(* Logix 5000 Program export Yaskawa_Ladder; software revision 17.00 *)

TYPE YaskawaParameters :   // DRIVE CONFIGURATION
STRUCT
   Parameters : DINT[43];   // DRIVE PARAMETERS
   Monitor : INT[43];   // DRIVE MONITOR VALUES
   CommsPath : STRING;   // COMMUNICATION PATH
   Slot : DINT;   // Slot # entered by HMI
   GetValues : BOOL;   // GET PARAMETER VALUES
   SetValues : BOOL;   // SET PARAMETER VALUES
   SetPath : BOOL;   // SET COMMUNICATIONS PATH
   MSG_Value : INT;   // INDIVIDUAL PARAMETER VALUE
   FinalFIFO_Pos : INT;   // FIFO LENGTH
   MSG_Attribute : INT;   // MESSAGE ATTRIBUTE CONFIGURATION
   MSG_Class : INT;   // MESSAGE CLASS CONFIGURATION
   MSG_Instance : INT;   // MESSAGE INSTANCE CONFIGURATION
   ONS : INT;   // ONE-SHOTS
   AttributeArray : INT[43];   // ATTRIBUTE ARRAY
   ClassArray : INT[43];   // CLASS ARRAY
   InstanceArray : INT[43];   // INSTANCE ARRAY
   CycleTimer : TIMER[7];   // MESSAGE TIMERS
   FIFO : CONTROL;   // PARAMETER FIFO
   Update : BOOL;   // GET MONITOR VALUES
   FIFO_Monitor : CONTROL;   // MONITOR FIFO
   MonitorMSG_Value : INT;   // INDIVIDUAL MONITOR VALUE
   Monitor_ClassArray : INT[43];   // MONITOR CLASS ARRAY
   Monitor_AttributeArray : INT[43];   // MONITOR ATTRIBUTE ARRAY
   Monitor_InstanceArray : INT[43];   // MONITOR INSTANCE ARRAY
   Monitor_MSG_Attribute : INT;   // MONITOR MESSAGE ATTRIBUTE CONFIGURATION
   Monitor_MSG_Class : INT;   // MONITOR MESSAGE CLASS CONFIGURATION
   Monitor_MSG_Instance : INT;   // MONITOR MESSAGE INSTANCE CONFIGURATION
   AB_CommsPath : STRING[17];   // AB SLOT CONFIG
   IP_StringCount : STRING[16];   // Indicates variable to use in path for given IP string character count
   MSG_CommsPath : STRING;   // TOTAL COMM PATH FOR MESSAGE INST
   counter : COUNTER[4];
   A : STRING;   // Constant string value A
   ASCII_Extract : DINT;
   B : STRING;   // Constant string value B
   C : STRING;   // Constant string value C
   Convert_Start : BOOL;   // Used to begin the convert of hex string to decimal value
   Current_Index : DINT;
   D : STRING;   // Constant string value D
   DINT : DINT;   // Holds value passed as input parameter from main routine
   E : STRING;   // Constant string value E
   EMPTY : STRING;   // Empty string used to reset the final string value before concatenation
   F : STRING;   // Constant string value F
   Hex_Entry_Flag : BOOL[32];   // Bit for HMI entry to trigger conversion of hex string to decimal
   Hex_OpEntry_Read : STRING[37];   // Array to hold hex string values for display on HMI
   Hex_OpEntry_Write : STRING[14];   // Array to hold hex string values entered by HMI to be converted
   Hex_Read_Placeholder : DINT;   // Placeholder to retrieve hex string for HMI display
   HTD_Number : DINT;
   HTD_String : STRING;
   J : DINT;   // Used to make a FOR/NEXT loop
   NUMBER : DINT;
   Partial_DINT : DINT[8];   // Holds individual parts from the original DINT values
   Partial_STRING : STRING[8];   // Holds individual from the original DINT in string format
   STRING : STRING;   // Contains the final value
   tempstring : STRING[4];   // Temporary string to concatinate communication path to message instructions
   Current_Fault : STRING;
   Last_Fault : STRING;
   Fault_Codes : STRING[775];
   K : DINT;
   Auto_Update : BOOL;   // Bit to turn on or off auto update of Monitor parameters
   MSGPath_Ending : STRING;   // Always $00
END_STRUCT
END_TYPE

VAR_GLOBAL   (* controller tags *)
   YaskawaMSG_Write : MESSAGE;   // YASKAWA DRIVE PARAMTER WRITE
        MessageParameters(MessageType := CIP Generic, RequestedLength := 2, ConnectedFlag := 2, ConnectionPath := test, 2, 192.165.1.165, ServiceCode := 16#0010, LocalElement := Yaskawa.MSG_Value)
   Yaskawa : YaskawaParameters;
        .PARAMETERS[1]   // DRIVE ENTRY PARAMETER
        .PARAMETERS[2]   // B1-01 - FREQUENCY REFERENCE SELECTION 1
        .PARAMETERS[3]   // B1-02 - RUN COMMAND SELECTION 1
        .PARAMETERS[4]   // C1-01 - ACCELERATION TIME
        .PARAMETERS[5]   // C1-02 - DECELERATION TIME
        .PARAMETERS[6]   // D1-01 - FREQUENCY REFERENCE 1
        .PARAMETERS[7]   // D1-02 - FREQUENCY REFERENCE 2
        .PARAMETERS[8]   // D1-03 - FREQUENCY REFERENCE 3
        .PARAMETERS[9]   // D1-04 - FREQUENCY REFERENCE 4
        .PARAMETERS[10]   // D1-17 - JOG REFERENCE
        .PARAMETERS[11]   // E1-01 - INPUT VOLTAGE
        .PARAMETERS[12]   // E1-04 - MAXIMUM OUTPUT FREQUENCY
        .PARAMETERS[13]   // E1-05 - MAXIMUM OUTPUT VOLTAGE
        .PARAMETERS[14]   // E1-06 - BASE FREQUENCY
        .PARAMETERS[15]   // E1-13 - BASE VOLTAGE
        .PARAMETERS[16]   // E2-01 - MOTOR RATED CURRENT
        .PARAMETERS[17]   // E2-02 - MOTOR RATED SLIP
        .PARAMETERS[18]   // E2-03 - MOTOR NO-LOAD CURRENT
        .PARAMETERS[19]   // E2-04 - NUMBER OF MOTOR POLES
        .PARAMETERS[20]   // E2-05 - MOTOR LINE TO LINE RESISTANCE
        .PARAMETERS[21]   // E2-11 - MOTOR RATED POWER
        .PARAMETERS[22]   // H1-01 - MULTI-FUNCTION INPUT S1
        .PARAMETERS[23]   // H1-02 - MULTI-FUNCTION INPUT S2
        .PARAMETERS[24]   // H1-03 - MULTI-FUNCTION INPUT S3
        .PARAMETERS[25]   // H1-04 - MULTI-FUNCTION INPUT S4
        .PARAMETERS[26]   // H1-05 - MULTI-FUNCTION INPUT S5
        .PARAMETERS[27]   // H1-06 - MULTI-FUNCTION INPUT S6
        .PARAMETERS[28]   // H1-07 - MULTI-FUNCTION INPUT S7
        .PARAMETERS[29]   // H1-08 - MULTI-FUNCTION INPUT S8
        .PARAMETERS[30]   // H2-01 - MULTI FUNCTION OUTPUT M1-M2
        .PARAMETERS[31]   // H2-02 - MULTI-FUNCTION OUTPUT M3-M4
        .PARAMETERS[32]   // H2-03 - MULTI FUNCTION OUTPUT M5-M6
        .PARAMETERS[33]   // H3-02 - TERMINAL A1 FUNCTION SELECTION
        .PARAMETERS[34]   // H3-06 - TERMINAL A3 FUNCTION SELECTION
        .PARAMETERS[35]   // H3-10 - TERMINAL A2 FUNCTION SELECTION
        .PARAMETERS[36]   // H4-01 - MULTI-FUNCTION ANALOG OUTPUT SELECTION (FM)
        .PARAMETERS[37]   // H4-04 - MULTI-FUNCTION ANALOG OUTPUT (AM)
        .PARAMETERS[38]   // L1-01 - MOTOR OVERLOAD PROTECTION SELECTION
        .PARAMETERS[39]   // L5-01 - NUMBER OF AUTO-RESTART ATTEMPTS
        .PARAMETERS[40]   // A1-02 - CONTROL METHOD
        .PARAMETERS[41]   // A1-06 - APPLICATION PRESETS
        .MONITOR[1]   // U1-02 - FREQUENCY OUTPUT
        .MONITOR[2]   // U1-03 - OUTPUT CURRENT
        .MONITOR[3]   // U1-05 - MOTOR SPEED
        .MONITOR[4]   // U1-06 - OUTPUT VOLTAGE
        .MONITOR[5]   // U1-07 - DC BUS VOLTAGE
        .MONITOR[6]   // U1-08 - OUTPUT POWER
        .MONITOR[7]   // U1-09 - TORQUE REFERENCE
        .MONITOR[8]   // U1-10 - INPUT TERMINAL STATUS
        .MONITOR[9]   // U1-11 - OUTPUT TERMINAL STATUS
        .MONITOR[10]   // U1-12 - DRIVE STATUS
        .MONITOR[11]   // U1-13 - TERMINAL A1 INPUT LEVEL
        .MONITOR[12]   // U1-14 - TERMINAL A2 INPUT LEVEL
        .MONITOR[13]   // U1-15 - TERMINAL A3 INPUT LEVEL
        .MONITOR[14]   // U2-01 - CURRENT FAULT
        .MONITOR[15]   // U2-02 - LAST FAULT
        .MONITOR[16]   // U2-03 - FREQUENCY REFERENCE AT PREVIOUS FAULT
        .MONITOR[17]   // U2-04 - OUTPUT FREQUENCY AT PREVIOUS FAULT
        .MONITOR[18]   // U2-05 - OUTPUT AT PREVIOUS FAULT
        .MONITOR[19]   // U2-06 - MOTOR SPEED AT PREVIOUS FAULT
        .MONITOR[20]   // U2-07 - OUTPUT VOLTAGE AT PREVIOUS FAULT
        .MONITOR[21]   // U2-08 - DC BUS VOLTAGE AT PREVIOUS FAULT
        .MONITOR[22]   // U2-09 - OUTPUT POWER AT PREVIOUS FAULT
        .MONITOR[23]   // U2-10 - TORQUE REFERENCE AT PREVIOUS FAULT
        .MONITOR[24]   // U2-11 - INPUT TERMINAL STATUS AT PREVIOUS FAULT
        .MONITOR[25]   // U2-12 - OUTPUT TERMINAL STATUS AT PREVIOUS FAULT
        .MONITOR[26]   // U2-13 - DRIVE OPERATION STATUS AT PREVIOUS FAULT
        .MONITOR[27]   // U2-14 - CUMULATIVE OPERATION TIME AT PREVIOUS FAULT
        .MONITOR[28]   // U1-01 - FREQUENCY REFERENCE
   YaskawaMSG_Monitor : MESSAGE;   // YASKAWA DRIVE MONITOR READ
        MessageParameters(MessageType := CIP Generic, ConnectedFlag := 2, ConnectionPath := test, 2, 192.165.1.165, ServiceCode := 16#000e, DestinationTag := Yaskawa.MonitorMSG_Value)
   YaskawaMSG_Read : MESSAGE;   // YASKAWA DRIVE PARAMETER READ
        MessageParameters(MessageType := CIP Generic, ConnectedFlag := 2, ConnectionPath := test, 2, 192.165.1.165, ServiceCode := 16#000e, DestinationTag := Yaskawa.MSG_Value)
END_VAR

PROGRAM Yaskawa_Ladder   (* main routine Yaskawa_Parameters *)

ROUTINE Yaskawa_Monitor   (* ladder *)
// Controls collecting U parameters for monitoring.
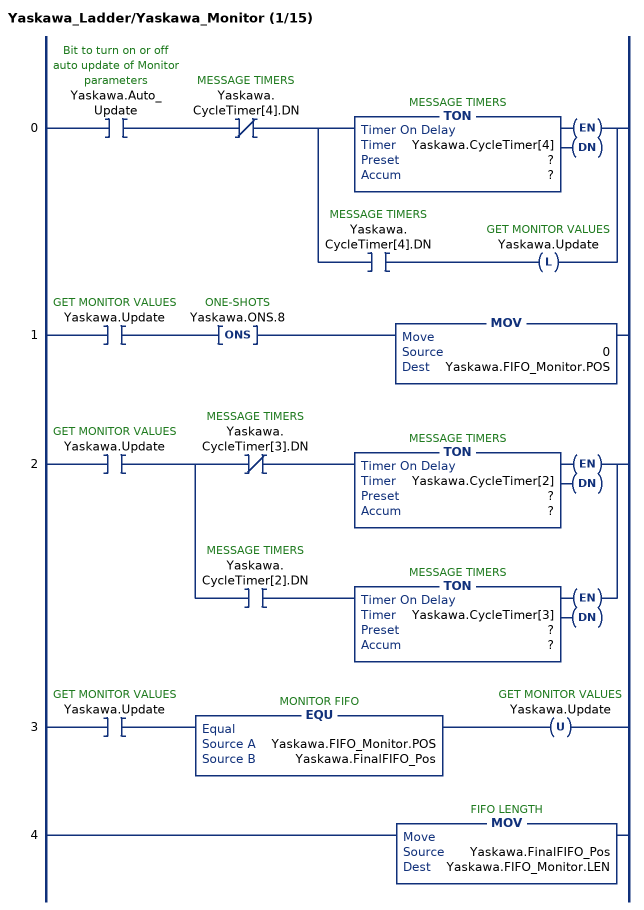
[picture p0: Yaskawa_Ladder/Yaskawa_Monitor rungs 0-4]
   0: XIC(Yaskawa.Auto_Update)XIO(Yaskawa.CycleTimer[4].DN)[TON(Yaskawa.CycleTimer[4],?,?) ,XIC(Yaskawa.CycleTimer[4].DN) OTL(Yaskawa.Update) ];
   1: XIC(Yaskawa.Update)ONS(Yaskawa.ONS.8)MOV(0,Yaskawa.FIFO_Monitor.POS);
   2: XIC(Yaskawa.Update)[XIO(Yaskawa.CycleTimer[3].DN) TON(Yaskawa.CycleTimer[2],?,?) ,XIC(Yaskawa.CycleTimer[2].DN) TON(Yaskawa.CycleTimer[3],?,?) ];
   3: XIC(Yaskawa.Update)EQU(Yaskawa.FIFO_Monitor.POS,Yaskawa.FinalFIFO_Pos)OTU(Yaskawa.Update);
   4: MOV(Yaskawa.FinalFIFO_Pos,Yaskawa.FIFO_Monitor.LEN);
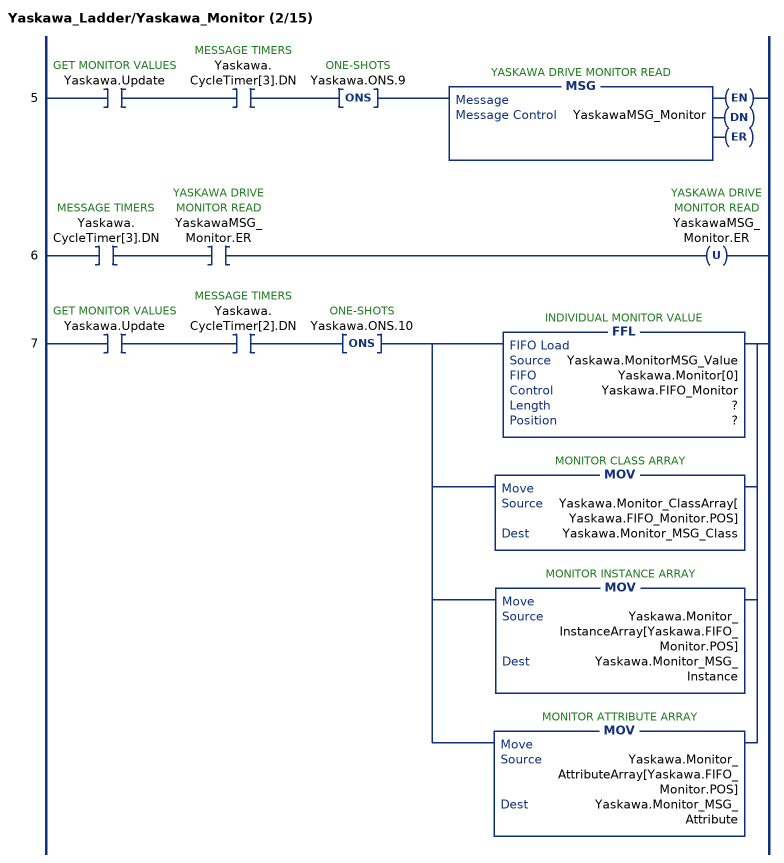
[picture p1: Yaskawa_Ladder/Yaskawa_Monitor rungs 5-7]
   5: XIC(Yaskawa.Update)XIC(Yaskawa.CycleTimer[3].DN)ONS(Yaskawa.ONS.9)MSG(YaskawaMSG_Monitor);
   6: XIC(Yaskawa.CycleTimer[3].DN)XIC(YaskawaMSG_Monitor.ER)OTU(YaskawaMSG_Monitor.ER);
   7: XIC(Yaskawa.Update)XIC(Yaskawa.CycleTimer[2].DN)ONS(Yaskawa.ONS.10)[FFL(Yaskawa.MonitorMSG_Value,Yaskawa.Monitor[0],Yaskawa.FIFO_Monitor,?,?) ,MOV(Yaskawa.Monitor_ClassArray[Yaskawa.FIFO_Monitor.POS],Yaskawa.Monitor_MSG_Class) ,MOV(Yaskawa.Monitor_InstanceArray[Yaskawa.FIFO_Monitor.POS],Yaskawa.Monitor_MSG_Instance) ,MOV(Yaskawa.Monitor_AttributeArray[Yaskawa.FIFO_Monitor.POS],Yaskawa.Monitor_MSG_Attribute) ];
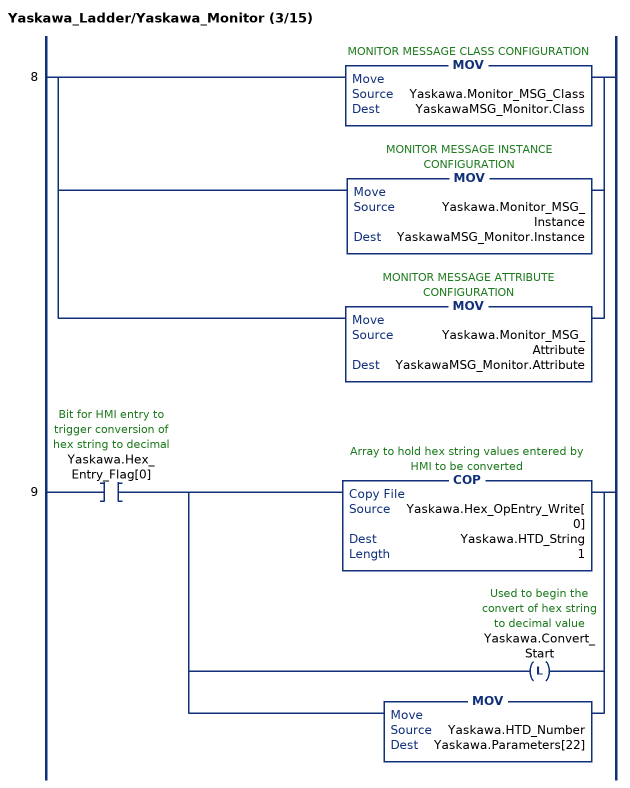
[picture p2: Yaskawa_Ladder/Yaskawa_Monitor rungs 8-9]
   8: [MOV(Yaskawa.Monitor_MSG_Class,YaskawaMSG_Monitor.Class) ,MOV(Yaskawa.Monitor_MSG_Instance,YaskawaMSG_Monitor.Instance) ,MOV(Yaskawa.Monitor_MSG_Attribute,YaskawaMSG_Monitor.Attribute) ];
   9: XIC(Yaskawa.Hex_Entry_Flag[0])[COP(Yaskawa.Hex_OpEntry_Write[0],Yaskawa.HTD_String,1) ,OTL(Yaskawa.Convert_Start) ,MOV(Yaskawa.HTD_Number,Yaskawa.Parameters[22]) ];
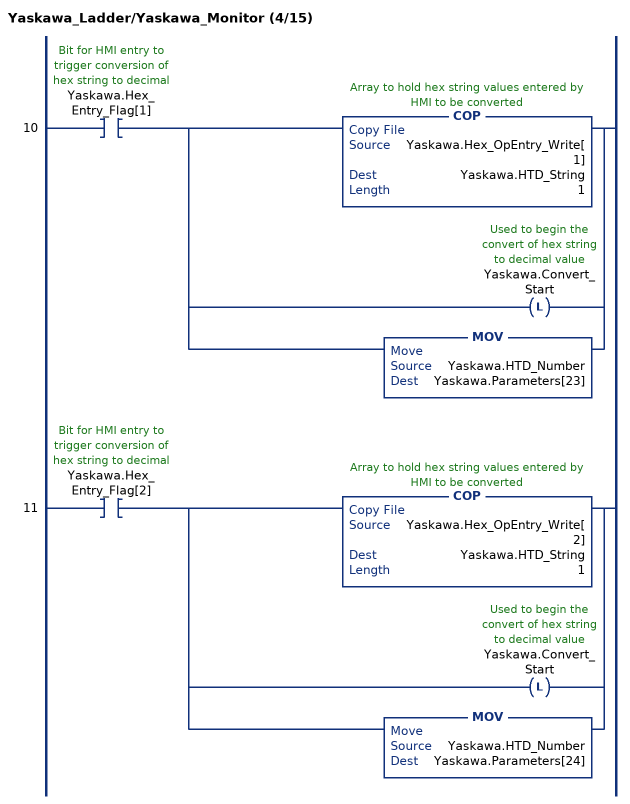
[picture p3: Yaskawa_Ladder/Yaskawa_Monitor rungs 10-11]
   10: XIC(Yaskawa.Hex_Entry_Flag[1])[COP(Yaskawa.Hex_OpEntry_Write[1],Yaskawa.HTD_String,1) ,OTL(Yaskawa.Convert_Start) ,MOV(Yaskawa.HTD_Number,Yaskawa.Parameters[23]) ];
   11: XIC(Yaskawa.Hex_Entry_Flag[2])[COP(Yaskawa.Hex_OpEntry_Write[2],Yaskawa.HTD_String,1) ,OTL(Yaskawa.Convert_Start) ,MOV(Yaskawa.HTD_Number,Yaskawa.Parameters[24]) ];
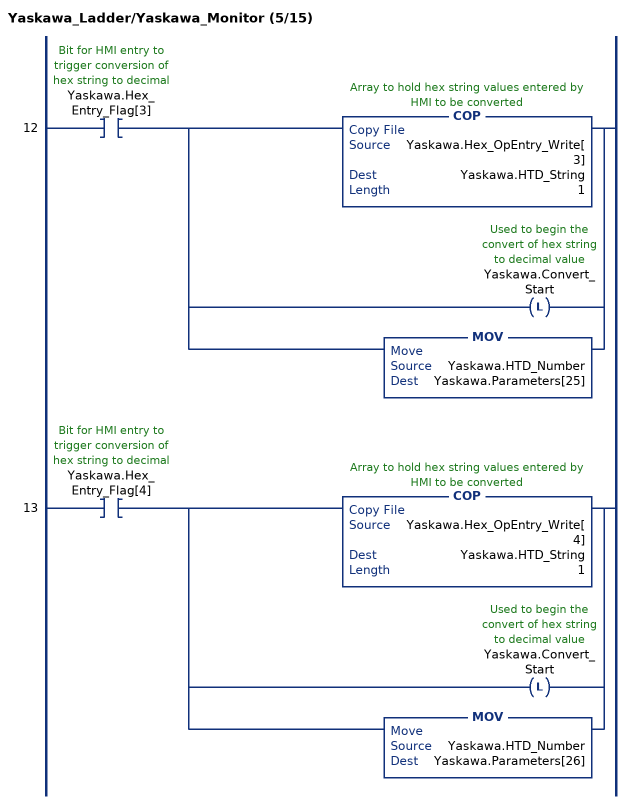
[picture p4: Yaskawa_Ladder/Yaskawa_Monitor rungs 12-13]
   12: XIC(Yaskawa.Hex_Entry_Flag[3])[COP(Yaskawa.Hex_OpEntry_Write[3],Yaskawa.HTD_String,1) ,OTL(Yaskawa.Convert_Start) ,MOV(Yaskawa.HTD_Number,Yaskawa.Parameters[25]) ];
   13: XIC(Yaskawa.Hex_Entry_Flag[4])[COP(Yaskawa.Hex_OpEntry_Write[4],Yaskawa.HTD_String,1) ,OTL(Yaskawa.Convert_Start) ,MOV(Yaskawa.HTD_Number,Yaskawa.Parameters[26]) ];
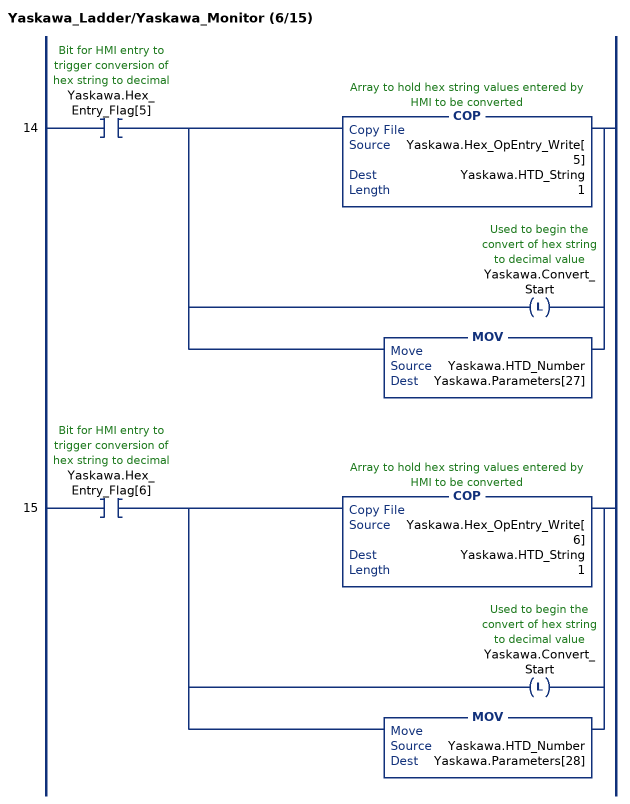
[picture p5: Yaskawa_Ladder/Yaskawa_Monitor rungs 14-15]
   14: XIC(Yaskawa.Hex_Entry_Flag[5])[COP(Yaskawa.Hex_OpEntry_Write[5],Yaskawa.HTD_String,1) ,OTL(Yaskawa.Convert_Start) ,MOV(Yaskawa.HTD_Number,Yaskawa.Parameters[27]) ];
   15: XIC(Yaskawa.Hex_Entry_Flag[6])[COP(Yaskawa.Hex_OpEntry_Write[6],Yaskawa.HTD_String,1) ,OTL(Yaskawa.Convert_Start) ,MOV(Yaskawa.HTD_Number,Yaskawa.Parameters[28]) ];
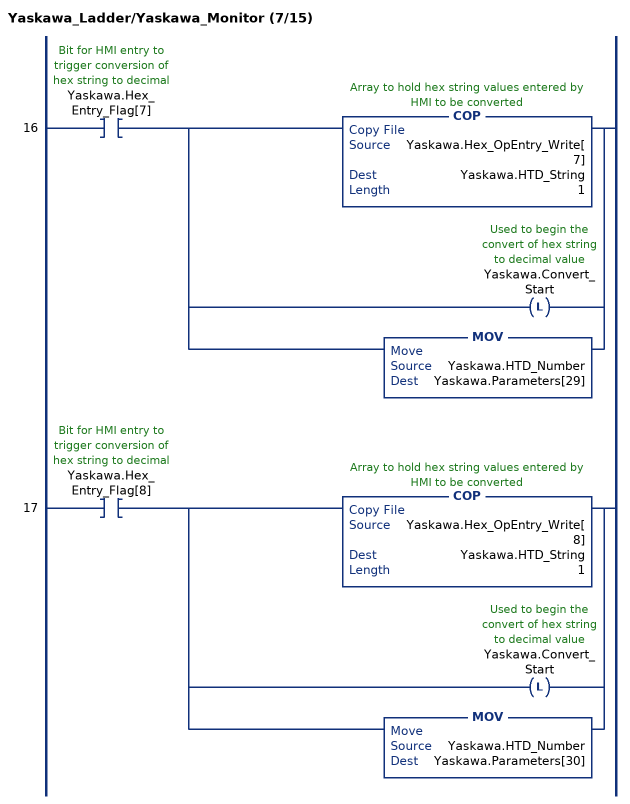
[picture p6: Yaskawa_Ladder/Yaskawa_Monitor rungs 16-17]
   16: XIC(Yaskawa.Hex_Entry_Flag[7])[COP(Yaskawa.Hex_OpEntry_Write[7],Yaskawa.HTD_String,1) ,OTL(Yaskawa.Convert_Start) ,MOV(Yaskawa.HTD_Number,Yaskawa.Parameters[29]) ];
   17: XIC(Yaskawa.Hex_Entry_Flag[8])[COP(Yaskawa.Hex_OpEntry_Write[8],Yaskawa.HTD_String,1) ,OTL(Yaskawa.Convert_Start) ,MOV(Yaskawa.HTD_Number,Yaskawa.Parameters[30]) ];
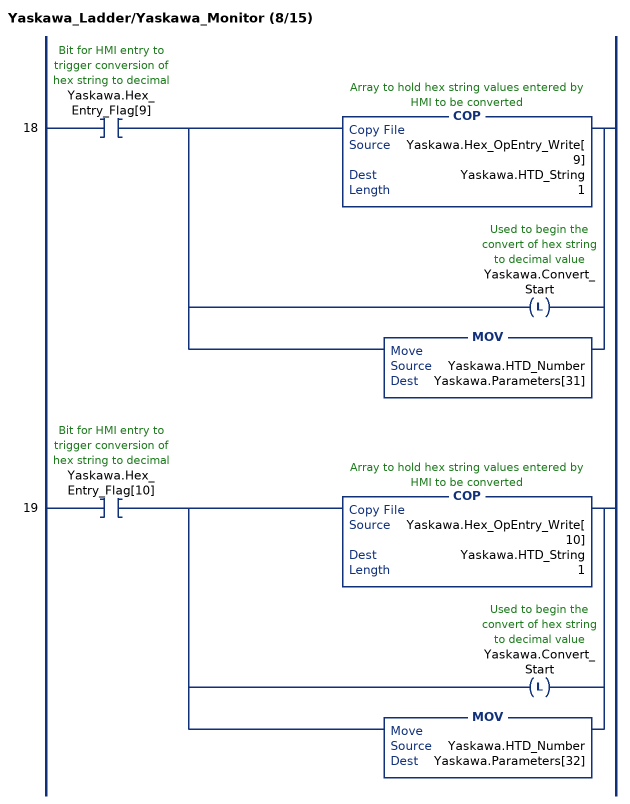
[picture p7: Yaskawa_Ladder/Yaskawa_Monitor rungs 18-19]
   18: XIC(Yaskawa.Hex_Entry_Flag[9])[COP(Yaskawa.Hex_OpEntry_Write[9],Yaskawa.HTD_String,1) ,OTL(Yaskawa.Convert_Start) ,MOV(Yaskawa.HTD_Number,Yaskawa.Parameters[31]) ];
   19: XIC(Yaskawa.Hex_Entry_Flag[10])[COP(Yaskawa.Hex_OpEntry_Write[10],Yaskawa.HTD_String,1) ,OTL(Yaskawa.Convert_Start) ,MOV(Yaskawa.HTD_Number,Yaskawa.Parameters[32]) ];
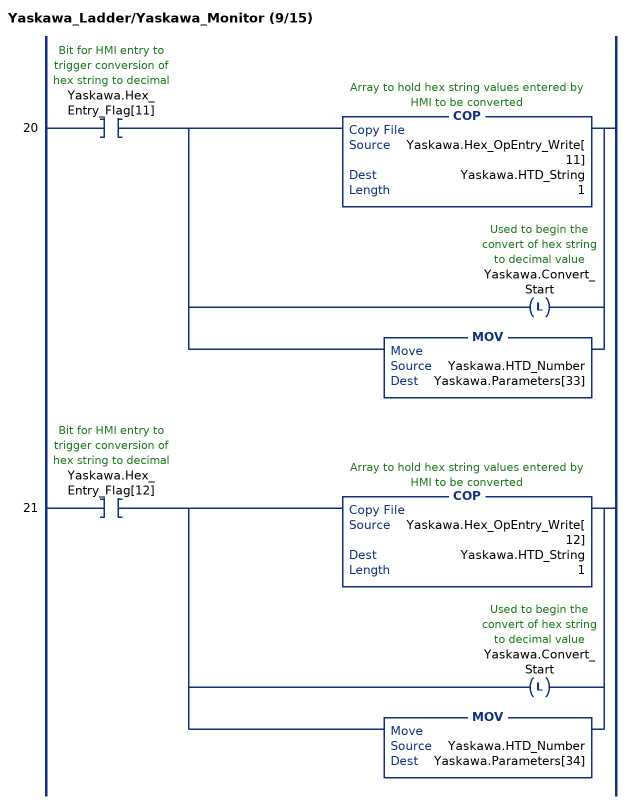
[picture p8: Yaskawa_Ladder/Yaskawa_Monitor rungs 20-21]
   20: XIC(Yaskawa.Hex_Entry_Flag[11])[COP(Yaskawa.Hex_OpEntry_Write[11],Yaskawa.HTD_String,1) ,OTL(Yaskawa.Convert_Start) ,MOV(Yaskawa.HTD_Number,Yaskawa.Parameters[33]) ];
   21: XIC(Yaskawa.Hex_Entry_Flag[12])[COP(Yaskawa.Hex_OpEntry_Write[12],Yaskawa.HTD_String,1) ,OTL(Yaskawa.Convert_Start) ,MOV(Yaskawa.HTD_Number,Yaskawa.Parameters[34]) ];
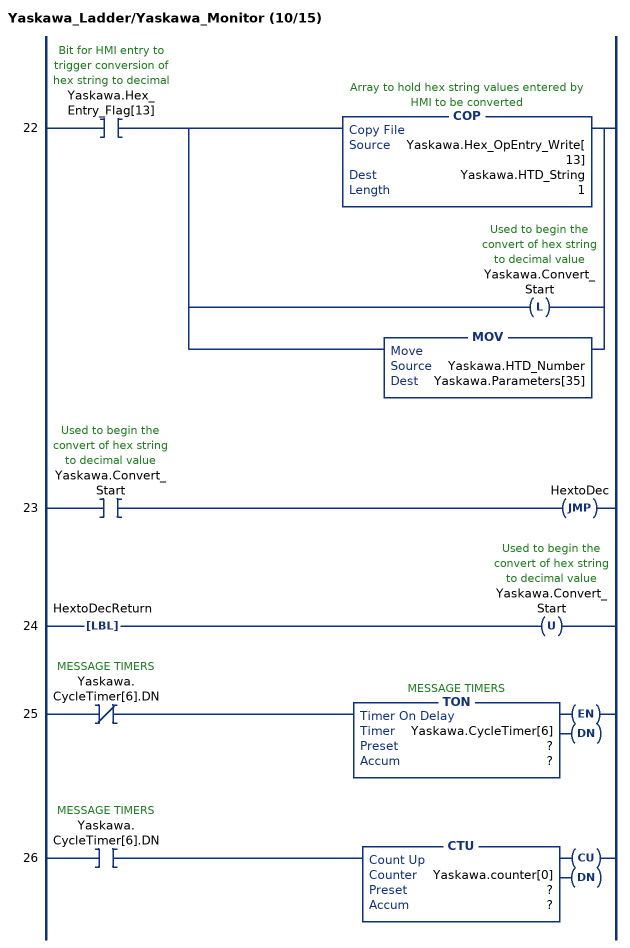
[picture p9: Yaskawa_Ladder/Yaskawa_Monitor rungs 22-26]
   22: XIC(Yaskawa.Hex_Entry_Flag[13])[COP(Yaskawa.Hex_OpEntry_Write[13],Yaskawa.HTD_String,1) ,OTL(Yaskawa.Convert_Start) ,MOV(Yaskawa.HTD_Number,Yaskawa.Parameters[35]) ];
   23: XIC(Yaskawa.Convert_Start)JMP(HextoDec);
   24: LBL(HextoDecReturn)OTU(Yaskawa.Convert_Start);
   25: XIO(Yaskawa.CycleTimer[6].DN)TON(Yaskawa.CycleTimer[6],?,?);
   26: XIC(Yaskawa.CycleTimer[6].DN)CTU(Yaskawa.counter[0],?,?);
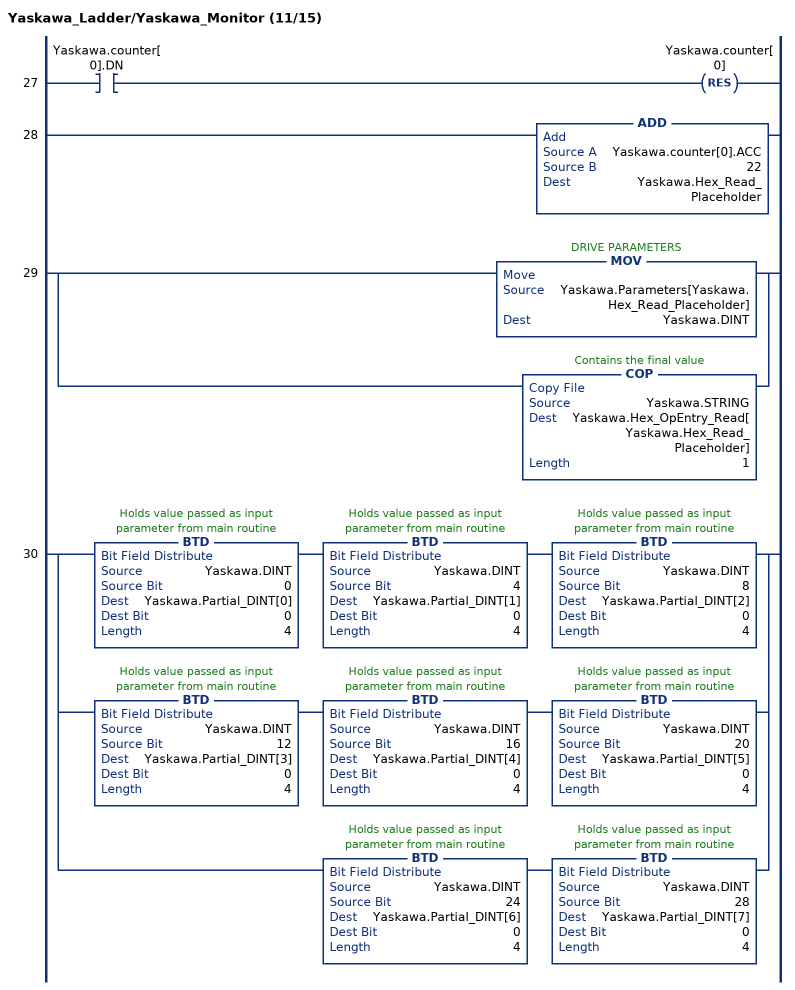
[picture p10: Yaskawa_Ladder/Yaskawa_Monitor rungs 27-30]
   27: XIC(Yaskawa.counter[0].DN)RES(Yaskawa.counter[0]);
   28: ADD(Yaskawa.counter[0].ACC,22,Yaskawa.Hex_Read_Placeholder);
   29: [MOV(Yaskawa.Parameters[Yaskawa.Hex_Read_Placeholder],Yaskawa.DINT) ,COP(Yaskawa.STRING,Yaskawa.Hex_OpEntry_Read[Yaskawa.Hex_Read_Placeholder],1) ];
   30: [BTD(Yaskawa.DINT,0,Yaskawa.Partial_DINT[0],0,4) BTD(Yaskawa.DINT,4,Yaskawa.Partial_DINT[1],0,4) BTD(Yaskawa.DINT,8,Yaskawa.Partial_DINT[2],0,4) ,BTD(Yaskawa.DINT,12,Yaskawa.Partial_DINT[3],0,4) BTD(Yaskawa.DINT,16,Yaskawa.Partial_DINT[4],0,4) BTD(Yaskawa.DINT,20,Yaskawa.Partial_DINT[5],0,4) ,BTD(Yaskawa.DINT,24,Yaskawa.Partial_DINT[6],0,4) BTD(Yaskawa.DINT,28,Yaskawa.Partial_DINT[7],0,4) ];
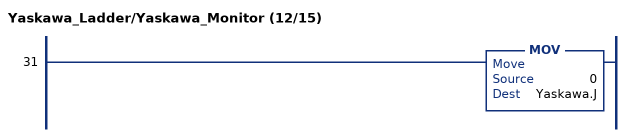
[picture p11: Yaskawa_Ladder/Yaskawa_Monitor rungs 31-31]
   31: MOV(0,Yaskawa.J);
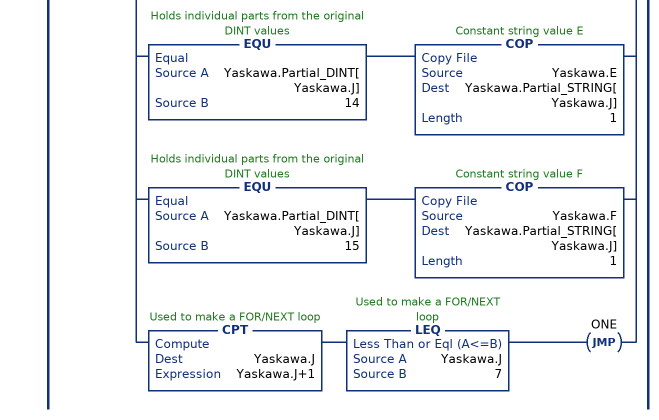
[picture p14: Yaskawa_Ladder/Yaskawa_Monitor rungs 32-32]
   32: LBL(ONE)[EQU(Yaskawa.Partial_DINT[Yaskawa.J],0) DTOS(Yaskawa.Partial_DINT[Yaskawa.J],Yaskawa.Partial_STRING[Yaskawa.J]) ,EQU(Yaskawa.Partial_DINT[Yaskawa.J],1) DTOS(Yaskawa.Partial_DINT[Yaskawa.J],Yaskawa.Partial_STRING[Yaskawa.J]) ,EQU(Yaskawa.Partial_DINT[Yaskawa.J],2) DTOS(Yaskawa.Partial_DINT[Yaskawa.J],Yaskawa.Partial_STRING[Yaskawa.J]) ,EQU(Yaskawa.Partial_DINT[Yaskawa.J],3) DTOS(Yaskawa.Partial_DINT[Yaskawa.J],Yaskawa.Partial_STRING[Yaskawa.J]) ,EQU(Yaskawa.Partial_DINT[Yaskawa.J],4) DTOS(Yaskawa.Partial_DINT[Yaskawa.J],Yaskawa.Partial_STRING[Yaskawa.J]) ,EQU(Yaskawa.Partial_DINT[Yaskawa.J],5) DTOS(Yaskawa.Partial_DINT[Yaskawa.J],Yaskawa.Partial_STRING[Yaskawa.J]) ,EQU(Yaskawa.Partial_DINT[Yaskawa.J],6) DTOS(Yaskawa.Partial_DINT[Yaskawa.J],Yaskawa.Partial_STRING[Yaskawa.J]) ,EQU(Yaskawa.Partial_DINT[Yaskawa.J],7) DTOS(Yaskawa.Partial_DINT[Yaskawa.J],Yaskawa.Partial_STRING[Yaskawa.J]) ,EQU(Yaskawa.Partial_DINT[Yaskawa.J],8) DTOS(Yaskawa.Partial_DINT[Yaskawa.J],Yaskawa.Partial_STRING[Yaskawa.J]) ,EQU(Yaskawa.Partial_DINT[Yaskawa.J],9) DTOS(Yaskawa.Partial_DINT[Yaskawa.J],Yaskawa.Partial_STRING[Yaskawa.J]) ,EQU(Yaskawa.Partial_DINT[Yaskawa.J],10) COP(Yaskawa.A,Yaskawa.Partial_STRING[Yaskawa.J],1) ,EQU(Yaskawa.Partial_DINT[Yaskawa.J],11) COP(Yaskawa.B,Yaskawa.Partial_STRING[Yaskawa.J],1) ,EQU(Yaskawa.Partial_DINT[Yaskawa.J],12) COP(Yaskawa.C,Yaskawa.Partial_STRING[Yaskawa.J],1) ,EQU(Yaskawa.Partial_DINT[Yaskawa.J],13) COP(Yaskawa.D,Yaskawa.Partial_STRING[Yaskawa.J],1) ,EQU(Yaskawa.Partial_DINT[Yaskawa.J],14) COP(Yaskawa.E,Yaskawa.Partial_STRING[Yaskawa.J],1) ,EQU(Yaskawa.Partial_DINT[Yaskawa.J],15) COP(Yaskawa.F,Yaskawa.Partial_STRING[Yaskawa.J],1) ,CPT(Yaskawa.J,Yaskawa.J+1) LEQ(Yaskawa.J,7) JMP(ONE) ];
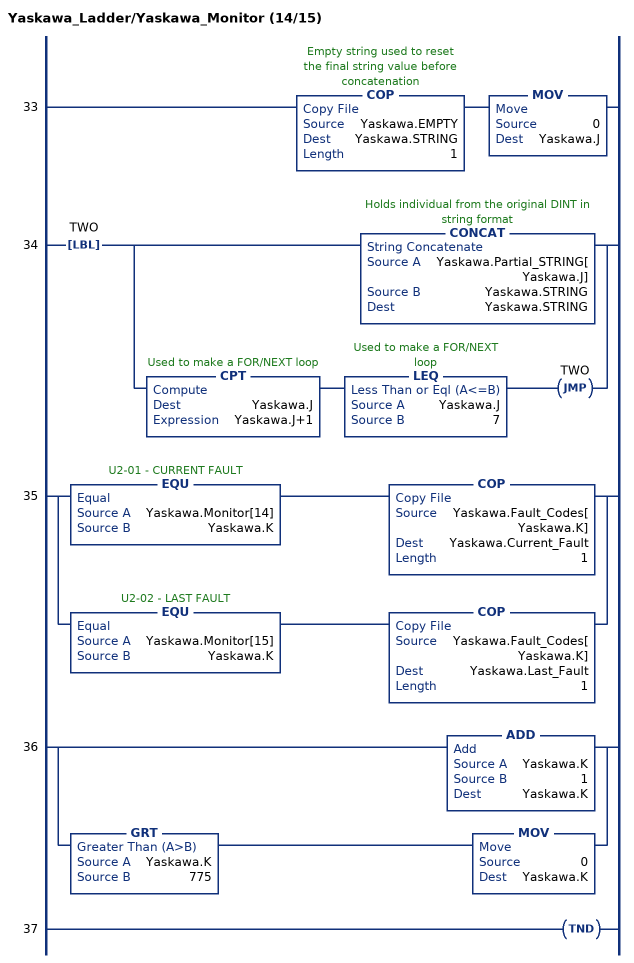
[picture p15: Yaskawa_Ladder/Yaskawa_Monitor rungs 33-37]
   33: COP(Yaskawa.EMPTY,Yaskawa.STRING,1)MOV(0,Yaskawa.J);
   34: LBL(TWO)[CONCAT(Yaskawa.Partial_STRING[Yaskawa.J],Yaskawa.STRING,Yaskawa.STRING) ,CPT(Yaskawa.J,Yaskawa.J+1) LEQ(Yaskawa.J,7) JMP(TWO) ];
   35: [EQU(Yaskawa.Monitor[14],Yaskawa.K) COP(Yaskawa.Fault_Codes[Yaskawa.K],Yaskawa.Current_Fault,1) ,EQU(Yaskawa.Monitor[15],Yaskawa.K) COP(Yaskawa.Fault_Codes[Yaskawa.K],Yaskawa.Last_Fault,1) ];
   36: [ADD(Yaskawa.K,1,Yaskawa.K) ,GRT(Yaskawa.K,775) MOV(0,Yaskawa.K) ];
   37: TND();
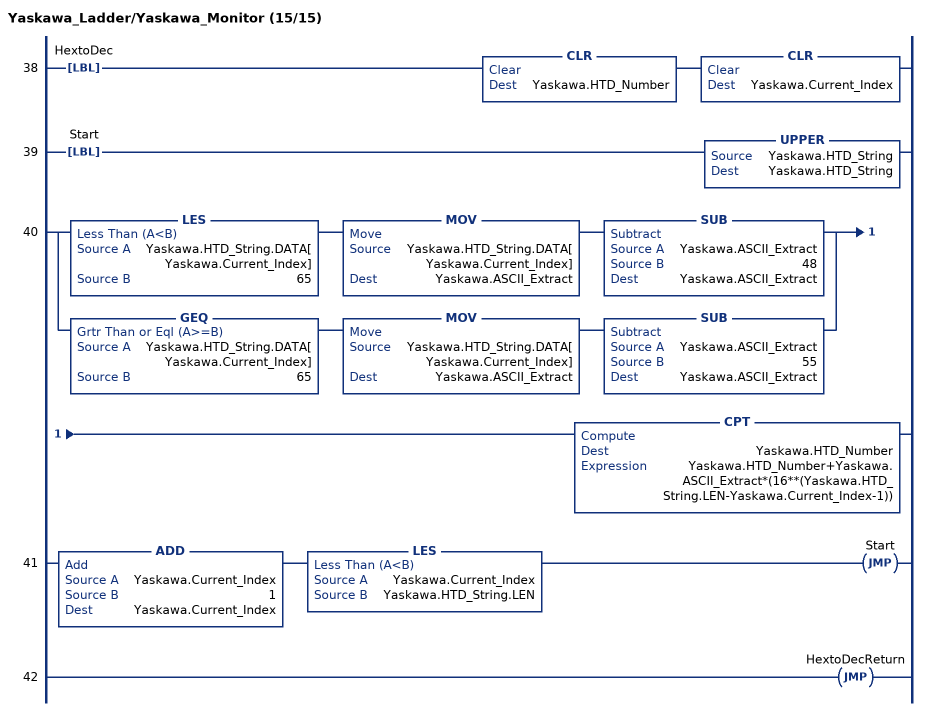
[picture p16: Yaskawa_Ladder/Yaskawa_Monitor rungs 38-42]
   38: LBL(HextoDec)CLR(Yaskawa.HTD_Number)CLR(Yaskawa.Current_Index);
   39: LBL(Start)UPPER(Yaskawa.HTD_String,Yaskawa.HTD_String);
   40: [LES(Yaskawa.HTD_String.DATA[Yaskawa.Current_Index],65) MOV(Yaskawa.HTD_String.DATA[Yaskawa.Current_Index],Yaskawa.ASCII_Extract) SUB(Yaskawa.ASCII_Extract,48,Yaskawa.ASCII_Extract) ,GEQ(Yaskawa.HTD_String.DATA[Yaskawa.Current_Index],65) MOV(Yaskawa.HTD_String.DATA[Yaskawa.Current_Index],Yaskawa.ASCII_Extract) SUB(Yaskawa.ASCII_Extract,55,Yaskawa.ASCII_Extract) ]CPT(Yaskawa.HTD_Number,Yaskawa.HTD_Number+Yaskawa.ASCII_Extract*(16**(Yaskawa.HTD_String.LEN-Yaskawa.Current_Index-1)));
   41: ADD(Yaskawa.Current_Index,1,Yaskawa.Current_Index)LES(Yaskawa.Current_Index,Yaskawa.HTD_String.LEN)JMP(Start);
   42: JMP(HextoDecReturn);
END_ROUTINE

ROUTINE Yaskawa_Parameters   (* ladder *)
// Controls reading and writing of parameters with PV+
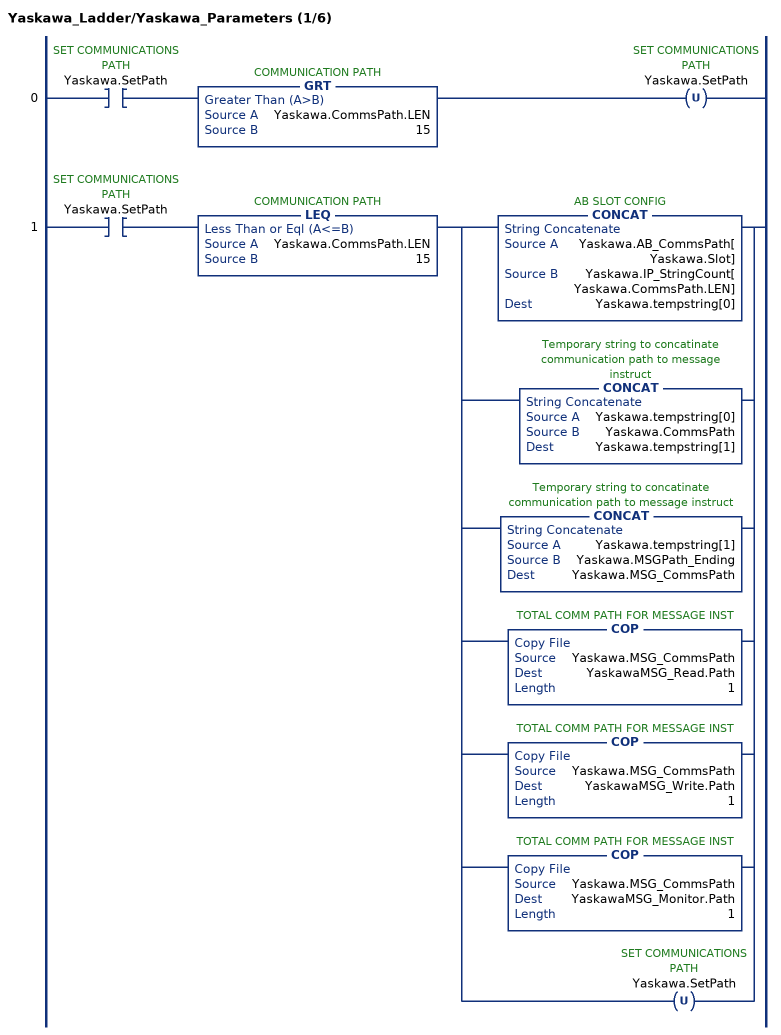
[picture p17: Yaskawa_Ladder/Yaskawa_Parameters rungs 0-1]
   0: XIC(Yaskawa.SetPath)GRT(Yaskawa.CommsPath.LEN,15)OTU(Yaskawa.SetPath);
   1: XIC(Yaskawa.SetPath)LEQ(Yaskawa.CommsPath.LEN,15)[CONCAT(Yaskawa.AB_CommsPath[Yaskawa.Slot],Yaskawa.IP_StringCount[Yaskawa.CommsPath.LEN],Yaskawa.tempstring[0]) ,CONCAT(Yaskawa.tempstring[0],Yaskawa.CommsPath,Yaskawa.tempstring[1]) ,CONCAT(Yaskawa.tempstring[1],Yaskawa.MSGPath_Ending,Yaskawa.MSG_CommsPath) ,COP(Yaskawa.MSG_CommsPath,YaskawaMSG_Read.Path,1) ,COP(Yaskawa.MSG_CommsPath,YaskawaMSG_Write.Path,1) ,COP(Yaskawa.MSG_CommsPath,YaskawaMSG_Monitor.Path,1) ,OTU(Yaskawa.SetPath) ];
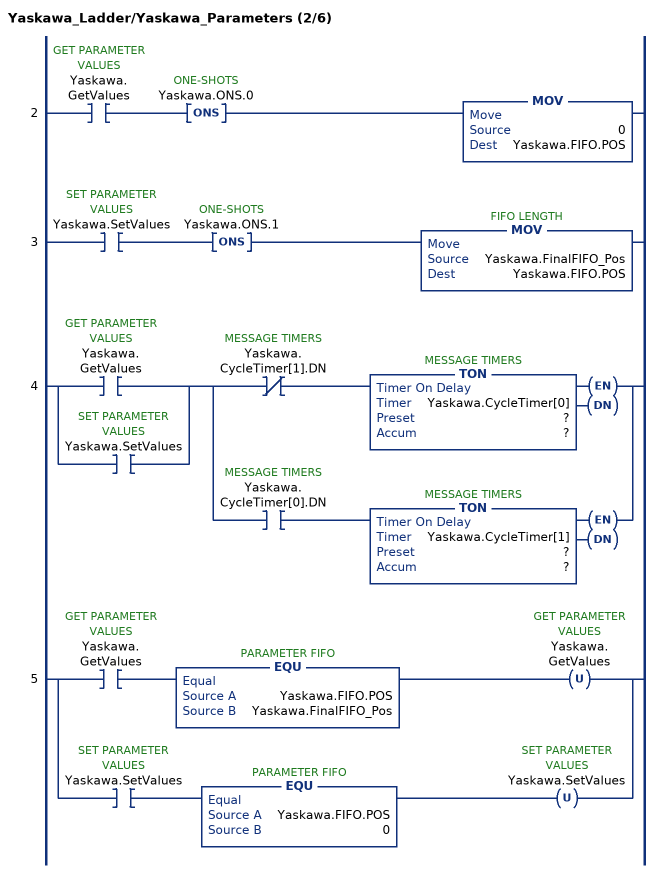
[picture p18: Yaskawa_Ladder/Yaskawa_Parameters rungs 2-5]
   2: XIC(Yaskawa.GetValues)ONS(Yaskawa.ONS.0)MOV(0,Yaskawa.FIFO.POS);
   3: XIC(Yaskawa.SetValues)ONS(Yaskawa.ONS.1)MOV(Yaskawa.FinalFIFO_Pos,Yaskawa.FIFO.POS);
   4: [XIC(Yaskawa.GetValues) ,XIC(Yaskawa.SetValues) ][XIO(Yaskawa.CycleTimer[1].DN) TON(Yaskawa.CycleTimer[0],?,?) ,XIC(Yaskawa.CycleTimer[0].DN) TON(Yaskawa.CycleTimer[1],?,?) ];
   5: [XIC(Yaskawa.GetValues) EQU(Yaskawa.FIFO.POS,Yaskawa.FinalFIFO_Pos) OTU(Yaskawa.GetValues) ,XIC(Yaskawa.SetValues) EQU(Yaskawa.FIFO.POS,0) OTU(Yaskawa.SetValues) ];
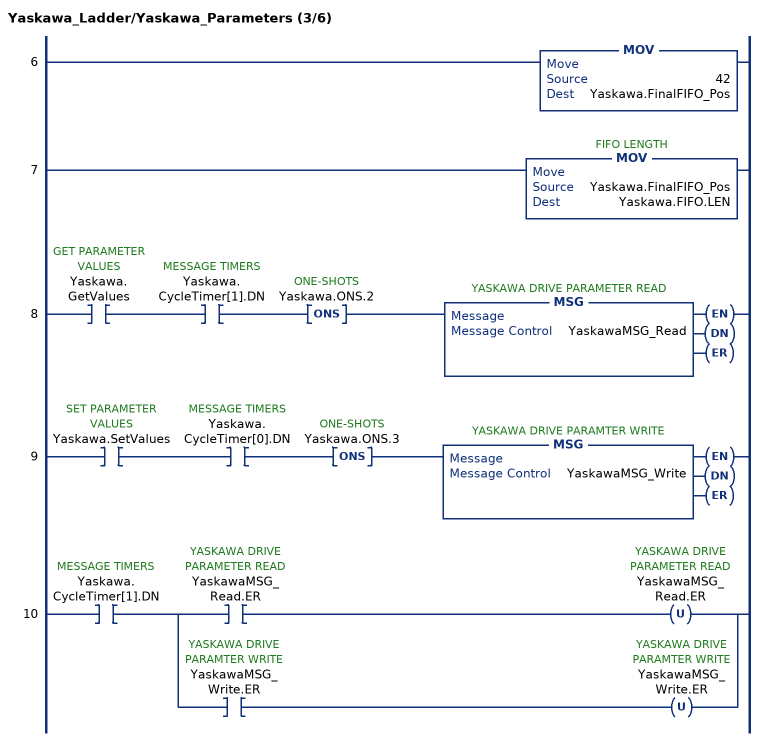
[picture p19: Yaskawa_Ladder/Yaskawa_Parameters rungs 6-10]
   6: MOV(42,Yaskawa.FinalFIFO_Pos);
   7: MOV(Yaskawa.FinalFIFO_Pos,Yaskawa.FIFO.LEN);
   8: XIC(Yaskawa.GetValues)XIC(Yaskawa.CycleTimer[1].DN)ONS(Yaskawa.ONS.2)MSG(YaskawaMSG_Read);
   9: XIC(Yaskawa.SetValues)XIC(Yaskawa.CycleTimer[0].DN)ONS(Yaskawa.ONS.3)MSG(YaskawaMSG_Write);
   10: XIC(Yaskawa.CycleTimer[1].DN)[XIC(YaskawaMSG_Read.ER) OTU(YaskawaMSG_Read.ER) ,XIC(YaskawaMSG_Write.ER) OTU(YaskawaMSG_Write.ER) ];
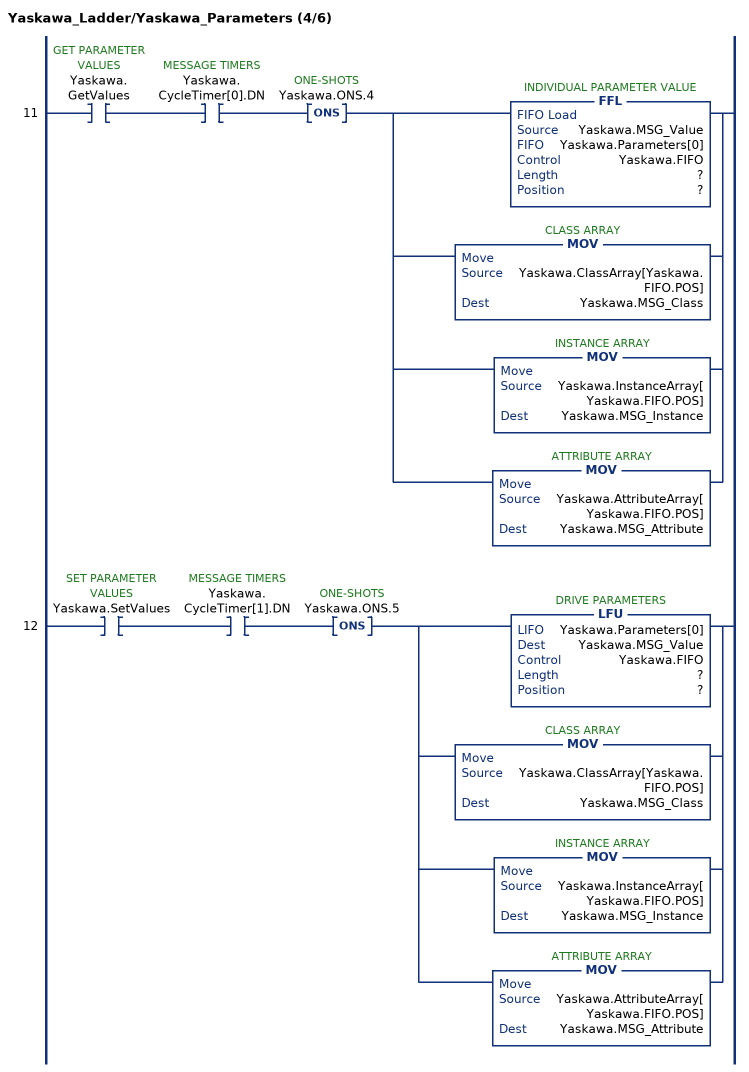
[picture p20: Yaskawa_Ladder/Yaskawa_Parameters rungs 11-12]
   11: XIC(Yaskawa.GetValues)XIC(Yaskawa.CycleTimer[0].DN)ONS(Yaskawa.ONS.4)[FFL(Yaskawa.MSG_Value,Yaskawa.Parameters[0],Yaskawa.FIFO,?,?) ,MOV(Yaskawa.ClassArray[Yaskawa.FIFO.POS],Yaskawa.MSG_Class) ,MOV(Yaskawa.InstanceArray[Yaskawa.FIFO.POS],Yaskawa.MSG_Instance) ,MOV(Yaskawa.AttributeArray[Yaskawa.FIFO.POS],Yaskawa.MSG_Attribute) ];
   12: XIC(Yaskawa.SetValues)XIC(Yaskawa.CycleTimer[1].DN)ONS(Yaskawa.ONS.5)[LFU(Yaskawa.Parameters[0],Yaskawa.MSG_Value,Yaskawa.FIFO,?,?) ,MOV(Yaskawa.ClassArray[Yaskawa.FIFO.POS],Yaskawa.MSG_Class) ,MOV(Yaskawa.InstanceArray[Yaskawa.FIFO.POS],Yaskawa.MSG_Instance) ,MOV(Yaskawa.AttributeArray[Yaskawa.FIFO.POS],Yaskawa.MSG_Attribute) ];
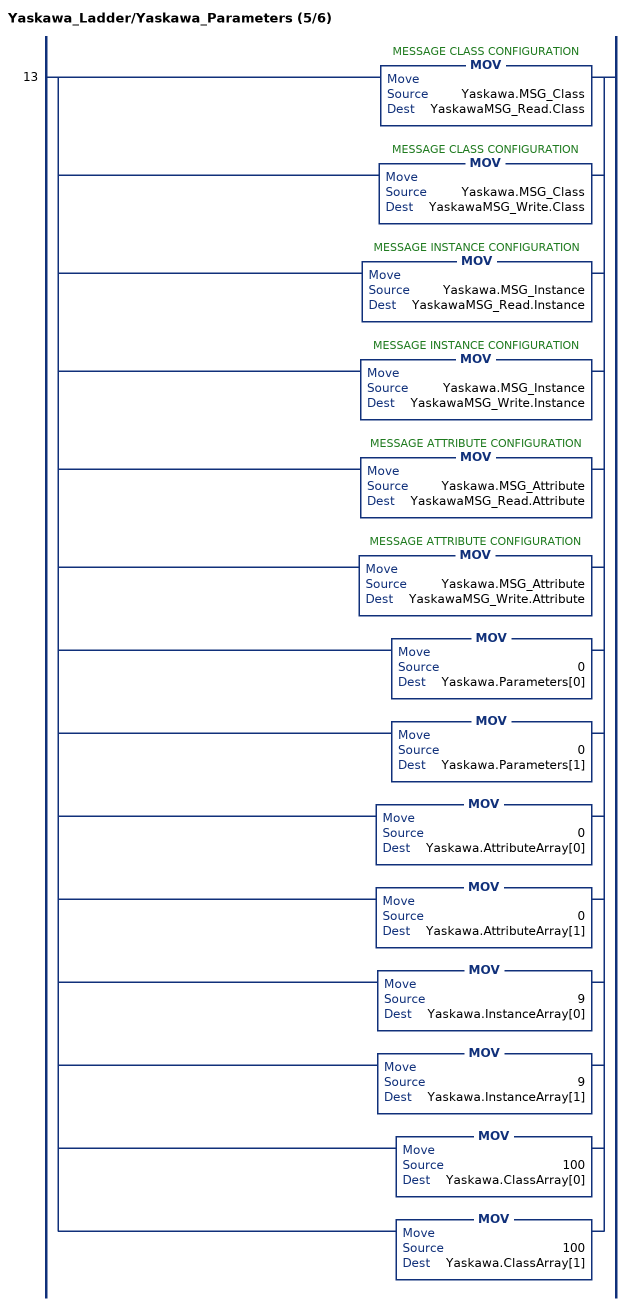
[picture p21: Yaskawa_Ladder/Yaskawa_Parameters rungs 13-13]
   13: [MOV(Yaskawa.MSG_Class,YaskawaMSG_Read.Class) ,MOV(Yaskawa.MSG_Class,YaskawaMSG_Write.Class) ,MOV(Yaskawa.MSG_Instance,YaskawaMSG_Read.Instance) ,MOV(Yaskawa.MSG_Instance,YaskawaMSG_Write.Instance) ,MOV(Yaskawa.MSG_Attribute,YaskawaMSG_Read.Attribute) ,MOV(Yaskawa.MSG_Attribute,YaskawaMSG_Write.Attribute) ,MOV(0,Yaskawa.Parameters[0]) ,MOV(0,Yaskawa.Parameters[1]) ,MOV(0,Yaskawa.AttributeArray[0]) ,MOV(0,Yaskawa.AttributeArray[1]) ,MOV(9,Yaskawa.InstanceArray[0]) ,MOV(9,Yaskawa.InstanceArray[1]) ,MOV(100,Yaskawa.ClassArray[0]) ,MOV(100,Yaskawa.ClassArray[1]) ];
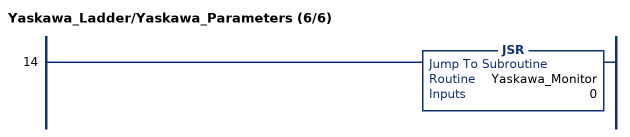
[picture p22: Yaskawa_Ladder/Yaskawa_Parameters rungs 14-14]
   14: JSR(Yaskawa_Monitor,0);
END_ROUTINE
END_PROGRAM
